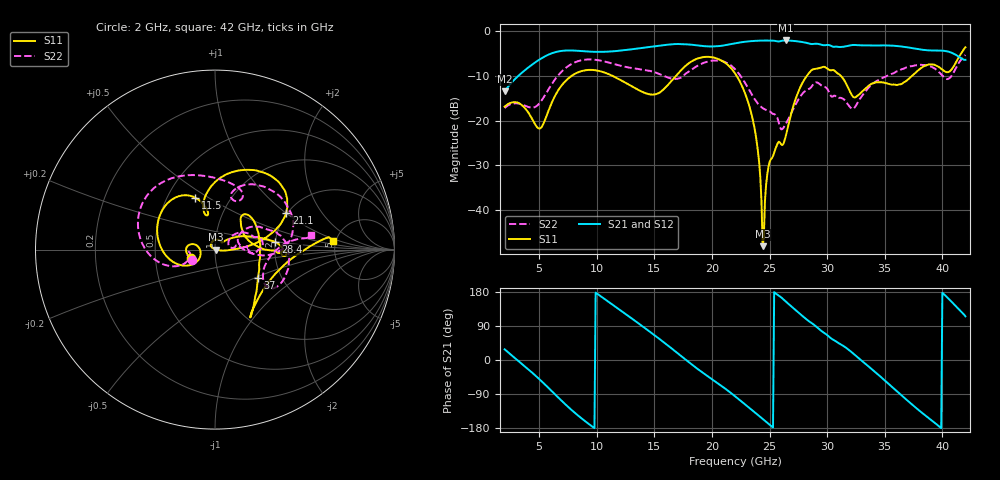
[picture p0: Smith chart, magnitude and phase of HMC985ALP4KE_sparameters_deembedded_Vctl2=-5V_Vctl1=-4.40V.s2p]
!s2p File: Measurements: S11, S21, S12, S22
# GHz S dB R 50.0
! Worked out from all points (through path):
!   401 points, 2 GHz to 42 GHz, reference 50 ohm
!   highest |S21| = -2.06 dB at 26.4 GHz (marker M1); lowest = -13.4 dB at 2 GHz (marker M2)
!   lowest |S11| = -48.0 dB at 24.4 GHz (marker M3), VSWR 1.01, Z = 50.4 + j0.0226 ohm
!   |S11| at or under -10 dB: start of sweep to 7.805 GHz; 22.15 GHz to 28.23 GHz (6.085 GHz wide, 24.2 % of centre); 31.19 GHz to 37.36 GHz (6.167 GHz wide, 18 % of centre)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
!   |S22| runs from -21.9 to -5.3 dB; largest |S21 - S12| = 0.00089
!   S11 on the Smith chart (normalised r, x): 2 GHz: 0.76, -0.07; 11.5 GHz: 0.68, +0.44; 21.1 GHz: 1.97, +1.02; 28.4 GHz: 2.00, +0.19; 37 GHz: 1.52, -0.52; 42 GHz: 4.77, +0.83
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2  -16.86 -161.7  -13.43 28.2  -13.44 28.2  -17.17 -155.6
5  -21.76 -172.6  -6.38 -50.1  -6.38 -50.1  -16.18 -159.9
6.3  -14.83 -150.4  -4.76 -88.3  -4.76 -88.3  -11.04 -161.6
8.7  -8.90 150.3  -4.44 -154.6  -4.44 -154.5  -6.47 151.3
11.5  -10.15 111.1  -4.47 143.1  -4.47 143.2  -7.33 105.1
13.6  -13.11 101.1  -3.85 97.2  -3.85 97.2  -8.44 75.8
15.4  -13.80 105.7  -3.25 56.5  -3.25 56.5  -9.53 62.4
17.9  -7.33 80.2  -2.94 -3.5  -2.94 -3.5  -9.16 72.3
21.1  -6.98 27.5  -3.14 -74.4  -3.14 -74.4  -6.87 16.1
22  -9.39 16.9  -2.71 -95.6  -2.71 -95.6  -8.47 0.7
23.6  -20.43 -0.2  -2.18 -135.3  -2.17 -135.3  -14.74 -3.9
24  -27.02 -7.3  -2.11 -145.3  -2.11 -145.3  -16.22 1.7
24.4  -48.05 3.2  -2.08 -155.4  -2.08 -155.4  -17.19 7.4
25  -29.27 133.3  -2.11 -170.7  -2.11 -170.7  -17.89 11.0
26.4  -23.51 42.7  -2.06 154.6  -2.06 154.6  -20.76 33.1
28.4  -9.41 7.2  -2.73 102.6  -2.73 102.7  -12.91 18.5
28.7  -8.60 2.1  -2.87 96.5  -2.87 96.5  -12.20 16.6
32.5  -14.69 33.0  -3.08 10.7  -3.08 10.8  -16.63 28.6
35.4  -11.79 19.1  -3.19 -64.7  -3.19 -64.7  -9.80 19.5
37  -10.83 -33.4  -3.62 -107.8  -3.62 -107.7  -8.02 5.1
39.8  -8.18 -56.8  -4.33 -177.3  -4.32 -177.2  -9.36 -34.9
42  -3.58 4.2  -6.39 115.2  -6.39 115.2  -5.32 8.9
